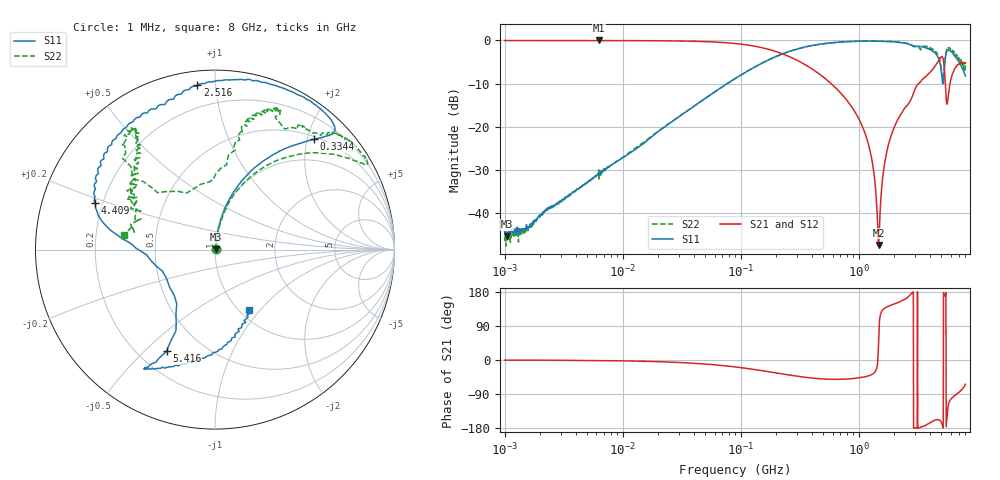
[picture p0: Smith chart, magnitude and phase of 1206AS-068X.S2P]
!s-Parameter Generated by FASTRON Sdn. Bhd.
!FASTRON P/N : 1206AS-068X
!Keysight Technologies: E5071C_MY46733604_B.14.02
!Date: Wed Nov 15 10:23:50 2023
!Version  :Rev00  Wed Nov 15 10:23:50 2023
!Data & Calibration Information:
!Freq  S11:SOLT2(ON)  S21:SOLT2(ON)  S12:SOLT2(ON)  S22:SOLT2(ON)
!PortZ  Port1:50+j0  Port2:50+j0
!When reading reference impedance value at option line is always used.
! Remarks : This data is being provided solely for informational purposes.
# Hz S dB R 50
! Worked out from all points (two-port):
!   1601 points, 1 MHz to 8 GHz, reference 50 ohm
!   highest |S21| = -0.02 dB at 6.301 MHz (marker M1); lowest = -47.3 dB at 1.473 GHz (marker M2)
!   |S21| within 3 dB of the highest: start of sweep to 221.3 MHz
!   lowest |S11| = -45.3 dB at 1.053 MHz (marker M3), VSWR 1.01, Z = 50.5 + j0.2 ohm
!   |S11| at or under -10 dB: start of sweep to 76.73 MHz; 5.14 GHz to 5.168 GHz (28.47 MHz wide, 0.552 % of centre)
!   |S22| runs from -47.6 to -0.1 dB; largest |S21 - S12| = 0.0065
!   S11 on the Smith chart (normalised r, x): 1 MHz: 1.01, +0.00; 334.4 MHz: 0.55, +2.13; 2.516 GHz: 0.07, +0.90; 4.409 GHz: 0.17, +0.18; 5.416 GHz: 0.31, -0.59; 8 GHz: 1.11, -0.87
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1000000  -44.26 19.9  -0.04 -0.4  -0.05 -0.3  -45.43 25.7
1052806  -45.35 21.5  -0.04 -0.4  -0.06 -0.3  -45.44 20.4
4479405  -33.72 73.9  -0.05 -1.0  -0.06 -1.0  -33.84 76.0
6301378  -30.94 72.1  -0.02 -1.5  -0.06 -1.5  -32.04 78.0
2.00676e7  -21.04 81.3  -0.09 -4.5  -0.11 -4.4  -20.97 80.7
8.994653e7  -8.79 70.9  -0.72 -18.3  -0.73 -18.3  -8.81 68.8
3.344081e8  -1.66 48.0  -5.29 -44.7  -5.30 -44.7  -1.66 40.4
4.006501e8  -1.20 46.1  -6.58 -47.5  -6.58 -47.5  -1.21 36.8
7.276733e8  -0.35 46.3  -12.64 -50.7  -12.65 -50.8  -0.37 29.7
1.064034e9  -0.18 53.5  -19.69 -45.8  -19.70 -45.9  -0.18 29.8
1.287677e9  -0.15 59.4  -27.41 -38.4  -27.42 -38.5  -0.14 31.3
1.473292e9  -0.21 65.1  -47.34 54.9  -47.38 54.8  -0.19 32.8
1.613809e9  -0.22 69.1  -30.50 133.7  -30.51 133.6  -0.21 34.0
1.7949e9  -0.29 74.5  -23.86 142.1  -23.87 141.9  -0.25 36.1
2.516241e9  -0.72 96.1  -15.26 162.1  -15.29 161.8  -0.62 43.6
3.466968e9  -1.55 128.6  -9.02 -176.0  -9.04 -176.0  -1.50 64.4
4.408619e9  -2.87 158.7  -6.07 -159.0  -6.06 -159.1  -2.36 74.7
5.052431e9  -8.36 -175.6  -3.75 -167.4  -3.72 -167.6  -7.43 89.2
5.416325e9  -4.05 -115.5  -10.30 170.3  -10.28 170.0  -3.62 135.4
5.668252e9  -2.28 -120.7  -13.91 -129.5  -13.89 -129.9  -1.82 128.6
6.149367e9  -2.76 -114.7  -8.18 -100.1  -8.16 -100.4  -2.09 124.4
8e9  -8.27 -60.5  -5.18 -64.1  -5.17 -64.6  -5.75 171.1
